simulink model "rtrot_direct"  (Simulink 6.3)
settings: Solver=ode45  SolverMode=SingleTasking  StartTime=0.0  StopTime=inf  FixedStep=h  RelTol=1e-3  AbsTol=1e-6
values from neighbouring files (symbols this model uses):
  adingain = [1.2*(pi*2/620/3)*[1 -1 -1 1 1 1] 1]    [hwinit.m]
  adinoffs = [-421 -511 -568 -518 -521 -410    0]    [hwinit.m]
  daoutgain = 127*[1 -1 -1 1 1 1 1]    [hwinit.m]
  daoutoffs = 127*[1 1 1 1 0.98 1 0]    [hwinit.m]
  h = 0.01    [design_pol.m]    (also in design_rot.m; design_wrist.m; rtrobot_init.m = 0.05; simpleregret.m = cfg.h)
  hc = 0.03    [design_pol.m]    (also in design_rot.m)
  joint = [1 2 3 4 5]    [design_pol.m]    (also in design_rot.m = [1 5]; design_wrist.m = [5]; rtrobot_init.m = joint(:)+(0:6:6*(n-1))')
  Kd = [0.4 0.1 0.1]    [design_pol.m]    (also in design_rot.m = [0.3 0.1]; design_wrist.m = 0.01; mc_approx_vectorized.m = cfg.Kd)
  Ki = [0.6 0.3 0.9]/3    [design_pol.m]    (also in design_rot.m = [0.1 0.1]; design_wrist.m = 0)
  Kp = [0.5 0.2 1.0]    [design_pol.m]    (also in design_rot.m = [0.4 2]; design_wrist.m = 1.5)
undefined symbols (not defined in the file or in its folder): COM1, DiscIntNeverNeededParam, No
libraries: simulink x5, xpclib x4, cstblocks x4, rtlib x1

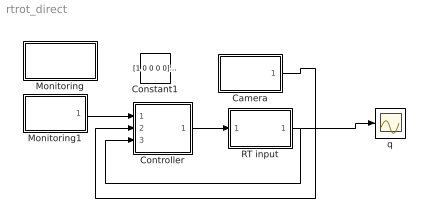
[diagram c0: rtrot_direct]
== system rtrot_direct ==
  Camera : Subsystem
  Constant1 : Constant  Value=[1 0 0 0 0]*pi/180*10
  Controller : Subsystem
  Monitoring : Subsystem
  Monitoring1 : Subsystem
  RT input : Subsystem  InitFcn=rtclear all  mask{h=h, joint=joint, Port=COM1, laser=No, gripper=No}
      mask prompts: h "Sample time [s]:"; joint "Joints to control (e.g., [1 2 4])"; Port "Serial port:"; laser "Enable laser input"; gripper "Enable gripper current sensor"
      mask init:
      | hwinit;
      | sen = joint(:);                             % read joint angles
      | if strcmp(gripper,'Yes'),                   % if gripper current desired
      |     sen = [sen; 7];                         % add to the list
      | end;    
      |                                             
      | n = length(sen);                            % number of sensors to be read
      | sen = sen+(0:7:7*(n-1))';                   % convert into sequential index
      | sen_select = zeros(7,n);                    % prepare zeros
      | sen_select(sen) = 1;                        % assign 1 at the right places
      | 
      | act = joint(:);                             % control joint actuators
      | if strcmp(laser,'Yes'),                     % if laser desired
      |     act = [act; 7];                         % add to the list
      | end;    
      |                                             
      | n = length(act);                            % number of actuators to be controlled
      | act = act+(0:7:7*(n-1))';                   % convert into sequential index
      | act_select = zeros(7,n);                    % prepare zeros
      | act_select(act) = 1;                        % assign 1 at the right places
  q : Scope
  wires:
  Monitoring1/1(r) -> Controller/1(r)
  Controller/1(out_1) -> RT input/1(Motors)
  Constant1/1 -> ?
  RT input/1(Angles) -> q/1, Controller/3(q)
  Camera/1(features) -> Controller/2(y)

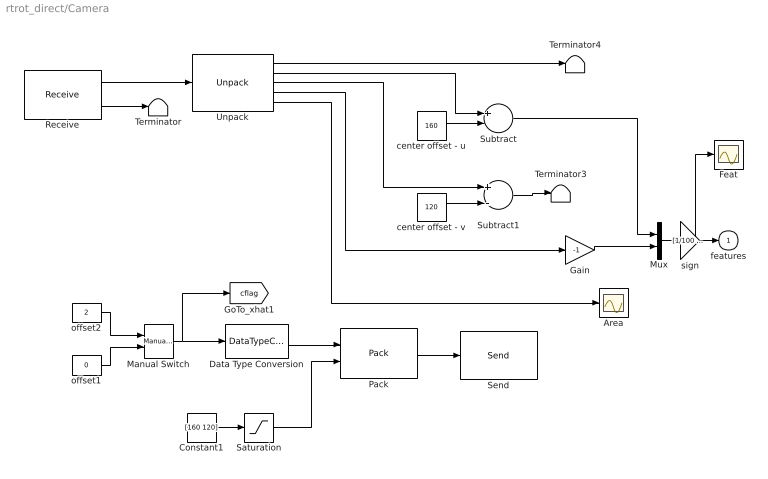
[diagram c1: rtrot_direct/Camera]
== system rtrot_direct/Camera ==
  Area : Scope
  Constant1 : Constant  Value=[160 120]
  Data Type Conversion : DataTypeConversion  OutDataTypeMode=uint8
  Feat : Scope
  Gain : Gain  Gain=-1
  Manual Switch : simulink/Signal Routing/Manual Switch  sw=1  action=0
  Mux : Mux  Inputs=2
  Pack : xpclib/UDP/Pack  datatypes={'uint8','double'}  byteAlign=4
  Receive : xpclib/UDP/Receive  ipAddress=127.0.0.1  ipPort=6907  width=40  sampletime=h
  Saturation : Saturate  UpperLimit=[320 240]  LowerLimit=[0 0]
  Send : xpclib/UDP/Send  ipAddress=127.0.0.1  ipPort=6906  localPort=-1  sampletime=h
  Subtract : Sum  Inputs=+-  OutScaling=2^-10
  Subtract1 : Sum  Inputs=+-  OutScaling=2^-10
  Terminator : Terminator
  Terminator3 : Terminator
  Terminator4 : Terminator
  Unpack : xpclib/UDP/Unpack  dimensions={1,1,1,1,1}  datatypes={'double','double','double','double','double'}  byteAlign=4
  center offset - u : Constant  Value=160
  center offset - v : Constant  Value=120
  offset1 : Constant  Value=0
  offset2 : Constant  Value=2
  sign : Gain  Gain=[1/100 1]  SampleTime=h
  features : Outport  InitialOutput=0
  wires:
  Receive/2 -> Terminator/1
  Receive/1 -> Unpack/1
  center offset - u/1 -> Subtract/2
  center offset - v/1 -> Subtract1/2
  Unpack/2 -> Subtract/1
  Unpack/3 -> Subtract1/1
  Unpack/4 -> Gain/1
  Subtract/1 -> Mux/1
  Unpack/5 -> Area/1
  Pack/1 -> Send/1
  Constant1/1 -> Saturation/1
  Data Type Conversion/1 -> Pack/1
  Saturation/1 -> Pack/2
  Subtract1/1 -> Terminator3/1
  Manual Switch/1 -> Data Type Conversion/1, [cflag]
  offset2/1 -> Manual Switch/1
  offset1/1 -> Manual Switch/2
  Mux/1 -> sign/1
  Unpack/1 -> Terminator4/1
  Gain/1 -> Mux/2
  sign/1 -> features/1, Feat/1

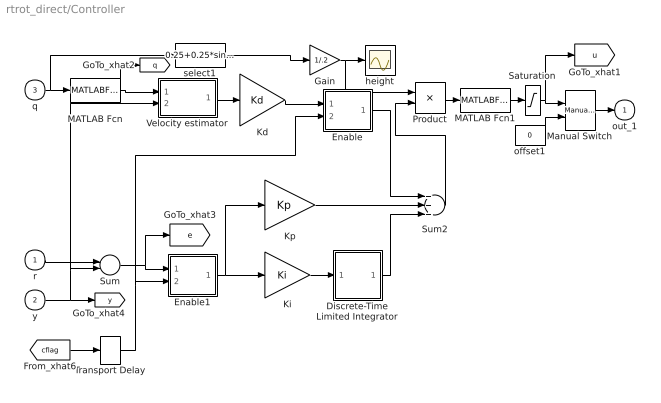
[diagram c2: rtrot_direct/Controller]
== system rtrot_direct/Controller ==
  r : Inport
  y : Inport  Port=2
  q : Inport  Port=3
  Discrete-Time Limited Integrator : Subsystem  mask(Discrete-Time Limited Integrator.){}
      mask help: Discrete-Time Limited Integrator.
      mask init:
      | lower_limit=@1;upper_limit=@2;X0=@3;Ts=@4;
  Enable : Subsystem
  Enable1 : Subsystem
  Gain : Gain  Gain=1/.2
  Kd : Gain  Gain=Kd  SampleTime=h
  Ki : Gain  Gain=Ki  SampleTime=h
  Kp : Gain  Gain=Kp  SampleTime=h
  MATLAB Fcn : MATLABFcn  MATLABFcn=[u(1) u(5)]
  MATLAB Fcn1 : MATLABFcn  MATLABFcn=[u(1) 0 0 0 u(2)]
  Manual Switch : simulink/Signal Routing/Manual Switch  sw=1  action=0
  Product : Product
  Saturation : Saturate  UpperLimit=[0.8 inf inf inf inf]  LowerLimit=[-0.8 -inf -inf -inf -inf]
  Sum : Sum  Inputs=+-  SampleTime=h
  Sum2 : Sum  Inputs=+++
  Transport Delay : TransportDelay  DelayTime=.1
  Velocity estimator : Subsystem
  height : Scope
  offset1 : Constant  Value=0
  select1 : Fcn  Expr=0.25+0.25*sin(u(2))+0.25*sin(u(2)+u(3))-0.15*cos(u(2)+u(3)+u(4))
  out_1 : Outport  InitialOutput=0
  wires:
  Discrete-Time Limited Integrator/1(out_1) -> Sum2/3
  Ki/1 -> Discrete-Time Limited Integrator/1(in_1)
  Enable1/1(Out) -> Ki/1, Kp/1
  Kp/1 -> Sum2/2
  r/1 -> Sum/1
  y/1 -> Velocity estimator/2(y), Sum/2, [y]
  Velocity estimator/1(v) -> Kd/1
  q/1 -> MATLAB Fcn/1, select1/1
  offset1/1 -> Manual Switch/2
  Manual Switch/1 -> out_1/1
  Sum/1 -> Enable1/1(In1), [e]
  Kd/1 -> Enable/1(In1)
  Enable/1(Out) -> Sum2/1
  [cflag] -> Transport Delay/1
  Transport Delay/1 -> Enable1/2(In2), Enable/2(In2)
  MATLAB Fcn/1 -> Velocity estimator/1(q), [q]
  select1/1 -> Gain/1
  Gain/1 -> height/1, Product/1
  Sum2/1 -> Product/2
  Product/1 -> MATLAB Fcn1/1
  MATLAB Fcn1/1 -> Saturation/1
  Saturation/1 -> Manual Switch/1, [u]

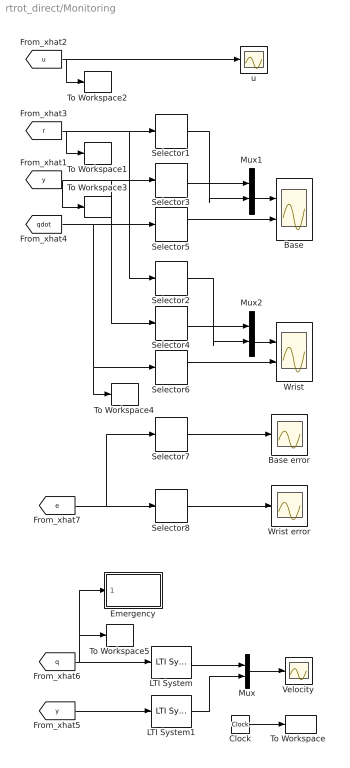
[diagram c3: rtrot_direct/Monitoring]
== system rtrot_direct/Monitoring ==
  Base : Scope  NumInputPorts=2
  Base error : Scope
  Clock : Clock
  Emergency : Subsystem
  LTI System : cstblocks/LTI System  sys=Gder  IC=[]
  LTI System1 : cstblocks/LTI System  sys=Gder  IC=[]
  Mux : Mux  Inputs=2
  Mux1 : Mux  Inputs=2
  Mux2 : Mux  Inputs=2
  Selector{1,3,5,7} (4 alike) : Selector  InputPortWidth=ny
  Selector{2,4,6,8} (4 alike) : Selector  Elements=2  InputPortWidth=ny
  "To Workspace  " : ToWorkspace  VariableName=t  SampleTime=h  SaveFormat=Array
  To Workspace1 : ToWorkspace  VariableName=r  SampleTime=h  SaveFormat=Array
  To Workspace2 : ToWorkspace  VariableName=u  SampleTime=h  SaveFormat=Array
  To Workspace3 : ToWorkspace  VariableName=y  SampleTime=h  SaveFormat=Array
  To Workspace4 : ToWorkspace  VariableName=qdot  SampleTime=h  SaveFormat=Array
  To Workspace5 : ToWorkspace  VariableName=q  SampleTime=h  SaveFormat=Array
  Velocity : Scope
  Wrist : Scope  NumInputPorts=2
  Wrist error : Scope
  u : Scope
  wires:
  Selector6/1 -> Wrist/2
  [u] -> u/1, To Workspace2/1
  [y] -> To Workspace3/1, Selector3/1, Selector4/1
  Mux1/1 -> Base/1
  [r] -> To Workspace1/1, Selector1/1, Selector2/1
  Clock/1 -> "To Workspace  "/1
  Mux2/1 -> Wrist/1
  Selector1/1 -> Mux1/2
  Selector2/1 -> Mux2/2
  Selector3/1 -> Mux1/1
  Selector4/1 -> Mux2/1
  [qdot] -> Selector5/1, Selector6/1, To Workspace4/1
  Selector5/1 -> Base/2
  Mux/1 -> Velocity/1
  LTI System/1 -> Mux/1
  LTI System1/1 -> Mux/2
  [y] -> LTI System1/1
  [q] -> LTI System/1, To Workspace5/1, Emergency/1(In1)
  Selector8/1 -> Wrist error/1
  [e] -> Selector8/1, Selector7/1
  Selector7/1 -> Base error/1

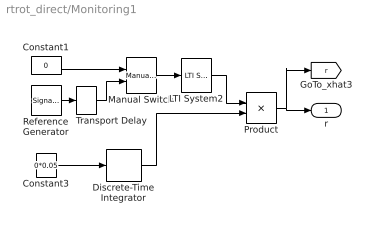
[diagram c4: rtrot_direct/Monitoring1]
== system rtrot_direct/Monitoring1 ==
  Constant1 : Constant  Value=0
  Constant3 : Constant  Value=0*0.05
  Discrete-Time Integrator : DiscreteIntegrator  InitialCondition=1  SampleTime=5  ICPrevOutput=DiscIntNeverNeededParam  ICPrevScaledInput=DiscIntNeverNeededParam
  LTI System2 : cstblocks/LTI System  sys=Fref  IC=[]
  Manual Switch : simulink/Signal Routing/Manual Switch  sw=1  action=0
  Product : Product
  Reference Generator : SignalGenerator  WaveForm=square  Amplitude=[0.4 0.3]  Frequency=1/5
  Transport Delay : TransportDelay  DelayTime=.5
  r : Outport
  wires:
  Product/1 -> r/1, [r]
  Constant3/1 -> Discrete-Time Integrator/1
  Discrete-Time Integrator/1 -> Product/2
  Manual Switch/1 -> LTI System2/1
  Reference Generator/1 -> Transport Delay/1
  Constant1/1 -> Manual Switch/1
  Transport Delay/1 -> Manual Switch/2
  LTI System2/1 -> Product/1

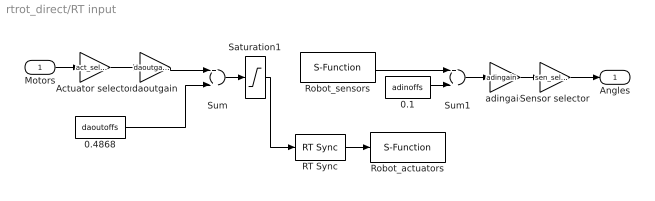
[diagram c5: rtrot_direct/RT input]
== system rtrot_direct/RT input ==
  Motors : Inport
  0.1 : Constant  Value=adinoffs
  0.4868 : Constant  Value=daoutoffs
  Actuator selector : Gain  Gain=act_select  Multiplication=Matrix(K*u)
  RT Sync : rtlib/RT Sync
  Robot_actuators : S-Function  FunctionName=sfserialout  Parameters=Ts, com  mask(Serial Out){Ts=h, Port=Port}
      mask prompts: Ts "Sample time:"; Port "Serial port:"
      mask help: Serial line output block
      mask init:
      | com = xserial('Port',Port,'Baudrate',115200);
  Robot_sensors : S-Function  FunctionName=sfserialin  Parameters=Ts, com  mask(Serial Out){Ts=h, Port=Port}
      mask prompts: Ts "Sample time:"; Port "Serial port:"
      mask help: Serial line output block
      mask init:
      | com = xserial('Port',Port,'Baudrate',115200);
  Saturation1 : Saturate  UpperLimit=255  LowerLimit=0
  Sensor selector : Gain  Gain=sen_select'  Multiplication=Matrix(K*u)
  Sum : Sum
  Sum1 : Sum
  adingain : Gain  Gain=adingain
  daoutgain : Gain  Gain=daoutgain
  Angles : Outport
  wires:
  RT Sync/1 -> Robot_actuators/1
  Actuator selector/1 -> daoutgain/1
  Sensor selector/1 -> Angles/1
  Saturation1/1 -> RT Sync/1
  daoutgain/1 -> Sum/1
  adingain/1 -> Sensor selector/1
  Robot_sensors/1 -> Sum1/1
  0.1/1 -> Sum1/2
  Sum1/1 -> adingain/1
  Motors/1 -> Actuator selector/1
  0.4868/1 -> Sum/2
  Sum/1 -> Saturation1/1

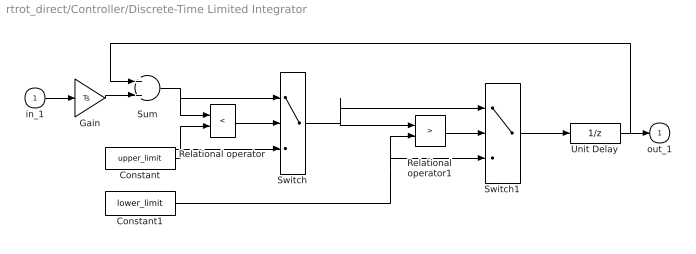
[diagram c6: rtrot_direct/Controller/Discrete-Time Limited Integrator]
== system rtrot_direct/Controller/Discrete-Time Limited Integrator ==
  in_1 : Inport
  Constant : Constant  Value=upper_limit
  Constant1 : Constant  Value=lower_limit
  Gain : Gain  Gain=Ts
  Relational operator : RelationalOperator  Operator=<
  Relational operator1 : RelationalOperator  Operator=>
  Sum : Sum
  Switch : Switch  Threshold=0.5
  Switch1 : Switch  Threshold=0.5
  Unit Delay : UnitDelay  X0=X0  SampleTime=Ts
  out_1 : Outport  InitialOutput=0
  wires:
  in_1/1 -> Gain/1
  Relational operator/1 -> Switch/2
  Sum/1 -> Relational operator/1, Switch/1
  Gain/1 -> Sum/2
  Constant/1 -> Relational operator/2, Switch/3
  Switch/1 -> Switch1/1, Relational operator1/1
  Relational operator1/1 -> Switch1/2
  Constant1/1 -> Switch1/3, Relational operator1/2
  Switch1/1 -> Unit Delay/1
  Unit Delay/1 -> Sum/1, out_1/1

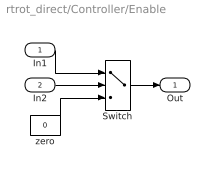
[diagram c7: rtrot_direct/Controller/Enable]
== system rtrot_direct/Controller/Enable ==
  In1 : Inport
  In2 : Inport  Port=2
  Switch : Switch  Threshold=0.5
  zero : Constant  Value=0
  Out : Outport
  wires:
  zero/1 -> Switch/3
  In2/1 -> Switch/2
  In1/1 -> Switch/1
  Switch/1 -> Out/1

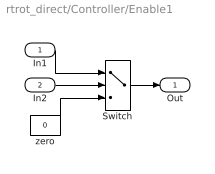
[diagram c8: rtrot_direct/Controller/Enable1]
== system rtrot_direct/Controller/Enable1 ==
  In1 : Inport
  In2 : Inport  Port=2
  Switch : Switch  Threshold=0.5
  zero : Constant  Value=0
  Out : Outport
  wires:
  zero/1 -> Switch/3
  In2/1 -> Switch/2
  In1/1 -> Switch/1
  Switch/1 -> Out/1

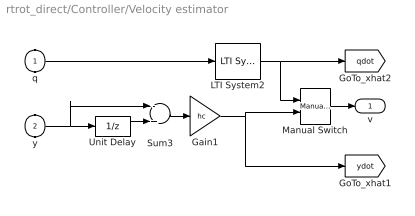
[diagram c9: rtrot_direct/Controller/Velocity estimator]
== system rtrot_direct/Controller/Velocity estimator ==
  q : Inport
  y : Inport  Port=2
  Gain1 : Gain  Gain=hc  SampleTime=hc
  LTI System2 : cstblocks/LTI System  sys=Gder1  IC=[]
  Manual Switch : simulink/Signal Routing/Manual Switch  sw=1  action=0
  Sum3 : Sum  Inputs=-+  SampleTime=h
  Unit Delay : UnitDelay  SampleTime=hc
  v : Outport
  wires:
  Unit Delay/1 -> Sum3/2
  Sum3/1 -> Gain1/1
  LTI System2/1 -> Manual Switch/1, [qdot]
  Gain1/1 -> Manual Switch/2, [ydot]
  y/1 -> Unit Delay/1, Sum3/1
  q/1 -> LTI System2/1
  Manual Switch/1 -> v/1

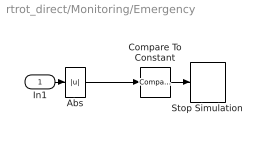
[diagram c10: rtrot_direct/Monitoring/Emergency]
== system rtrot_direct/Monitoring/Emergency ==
  In1 : Inport
  Abs : Abs
  Compare To Constant : simulink/Logic and Bit Operations/Compare To Constant  relop=>  const=[0.8 inf]  LogicOutDataTypeMode=boolean  ZeroCross=off
  Stop Simulation : Stop
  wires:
  Abs/1 -> Compare To Constant/1
  Compare To Constant/1 -> Stop Simulation/1
  In1/1 -> Abs/1
